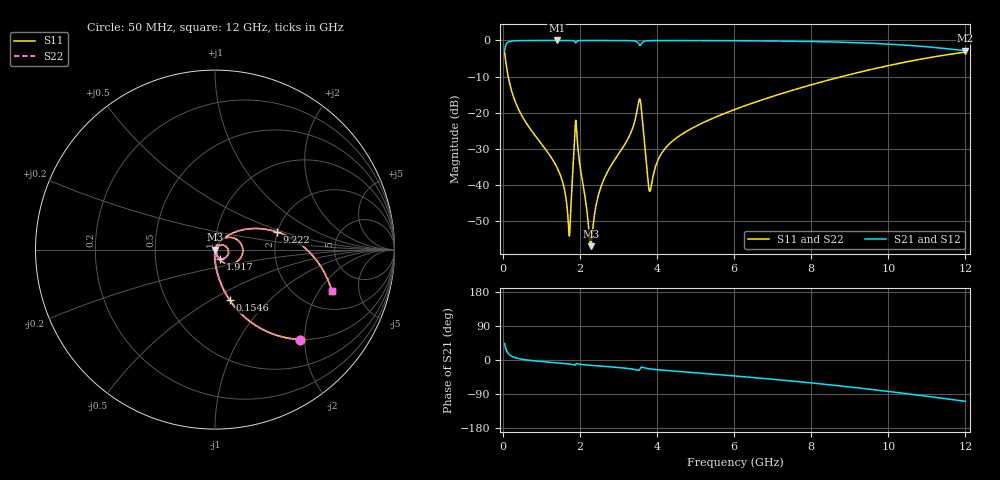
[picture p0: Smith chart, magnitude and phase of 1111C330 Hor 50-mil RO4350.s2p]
# GHz S MA R 50
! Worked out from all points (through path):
!   1601 points, 50 MHz to 12 GHz, reference 50 ohm
!   highest |S21| = -0.01 dB at 1.402 GHz (marker M1); lowest = -2.9 dB at 12 GHz (marker M2)
!   group delay of S21, straight-line fit = 25.7 ps
!   lowest |S11| = -56.9 dB at 2.283 GHz (marker M3), VSWR 1.00, Z = 50.1 - j0.029 ohm
!   |S11| at or under -10 dB: 142.9 MHz to 8.795 GHz (8.652 GHz wide, 194 % of centre)
!   |S22| runs from -56.9 to -3.2 dB; largest |S21 - S12| = 0
!   S11 on the Smith chart (normalised r, x): 50 MHz: 0.99, -1.90; 154.6 MHz: 0.99, -0.61; 1.917 GHz: 1.06, -0.11; 9.222 GHz: 1.99, +0.45; 12 GHz: 3.00, -2.62
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0.05  0.6911 -46.6  0.7226 43.4  0.7226 43.4  0.6911 -46.6
0.1545625  0.2943 -73.8  0.9554 16.2  0.9554 16.2  0.2943 -73.8
0.4831875  0.09382 -87.3  0.995 2.4  0.995 2.4  0.09382 -87.3
1.401844  0.01772 -94.8  0.9989 -7.6  0.9989 -7.6  0.01772 -94.8
1.723  0.002035 -34.7  0.998 -10.5  0.998 -10.5  0.002035 -34.7
1.775281  0.005778 47.2  0.9968 -11.2  0.9968 -11.2  0.005778 47.2
1.857438  0.03548 42.1  0.9792 -13.1  0.9792 -13.1  0.03548 42.1
1.917188  0.05794 -59.4  0.9618 -9.2  0.9618 -9.2  0.05794 -59.4
2.044156  0.0135 -89.7  0.997 -11.8  0.997 -11.8  0.0135 -89.7
2.283156  0.001424 -11.7  0.9984 -14.0  0.9984 -14.0  0.001424 -11.7
2.566969  0.01002 65.9  0.9984 -16.3  0.9984 -16.3  0.01002 65.9
3.291437  0.04827 61.0  0.9935 -22.8  0.9935 -22.8  0.04827 61.0
3.530438  0.145 15.9  0.889 -27.2  0.889 -27.2  0.145 15.9
3.597656  0.1115 -45.8  0.899 -19.0  0.899 -19.0  0.1115 -45.8
3.806781  0.008217 -12.6  0.9917 -23.2  0.9917 -23.2  0.008217 -12.6
4.038312  0.02277 55.3  0.996 -25.8  0.996 -25.8  0.02277 55.3
4.635813  0.04997 56.7  0.9963 -30.8  0.9963 -30.8  0.04997 56.7
6.025  0.1112 46.7  0.9913 -42.2  0.9913 -42.2  0.1112 46.7
8.019156  0.2448 28.7  0.9662 -60.6  0.9662 -60.6  0.2448 28.7
9.221625  0.3602 15.8  0.9287 -73.6  0.9287 -73.6  0.3602 15.8
10.01331  0.4496 6.4  0.8885 -83.1  0.8885 -83.1  0.4496 6.4
12  0.6897 -19.5  0.7178 -109.0  0.7178 -109.0  0.6897 -19.5
